(* Logix 5000 AddOnInstructionDefinition export AMCI_SV160E2_Tuning; software revision 20.03 *)

ADD_ON_INSTRUCTION AMCI_SV160E2_Tuning   (* revision 1.0, vendor AMCI, ExecuteEnableInFalse *)
// Revision note:
// 8/2019 Version 0 Initial release of SV160E2 Add On Instructions.
// 3/17/20 Version 1 replaced the generic EDS file with a more complete V1.6 EDS file.
VAR_INPUT
   Status_Word_0 : INT; {required}
        .0   // Set when the SV160E2 is moving CW
        .1   // Set when SV160E2 is moving CCW
        .7   // SV160E2 Move Complete bit
        .11   // Set when there is an input error
        .12   // set when there is a command error
        .13   // set when there is a configuration error
   Status_Word_1 : INT; {required}
        .15   // Set when SV160E2 is enabled
   Veloctiy_Loop_Proportional_Gain : INT; {required}
   Velocity_Loop_Integral_Gain : INT; {required}
   Velocity_Feedback_Low_Pass_Filter : INT; {required}
   Position_Loop_Proportional_Gain : INT; {required}
   Position_Loop_Integral_Gain : INT; {required}
   Position_Loop_Derivative_Gain : INT; {required}
   Maximim_Position_Error_Limit : INT; {required}
END_VAR
VAR_IN_OUT
   AMCI_SV160E2_output_data : _000A:SV160E2_9125ACD4:O:0; {required}
END_VAR
VAR_OUTPUT
   EN : BOOL; {access Read Only, visible}   // AOI EN bit
   DN : BOOL; {access Read Only, visible}   // AOI DN bit
   Config_ER : BOOL; {access Read Only, visible}   // AOI ER bit
   data_block_with_error : INT; {access Read Only, visible}
   data_word_with_error : INT; {access Read Only, visible}
END_VAR
VAR
   command_data_block : INT[10];
   tuning_counter : COUNTER := (PRE := 2); {access None}
END_VAR

ROUTINE EnableInFalse   (* ladder *)
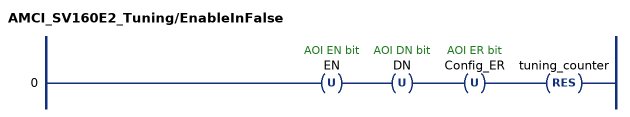
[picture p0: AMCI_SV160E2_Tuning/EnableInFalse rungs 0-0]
   0: OTU(EN)OTU(DN)OTU(Config_ER)RES(tuning_counter);
END_ROUTINE

ROUTINE Logic   (* ladder *)
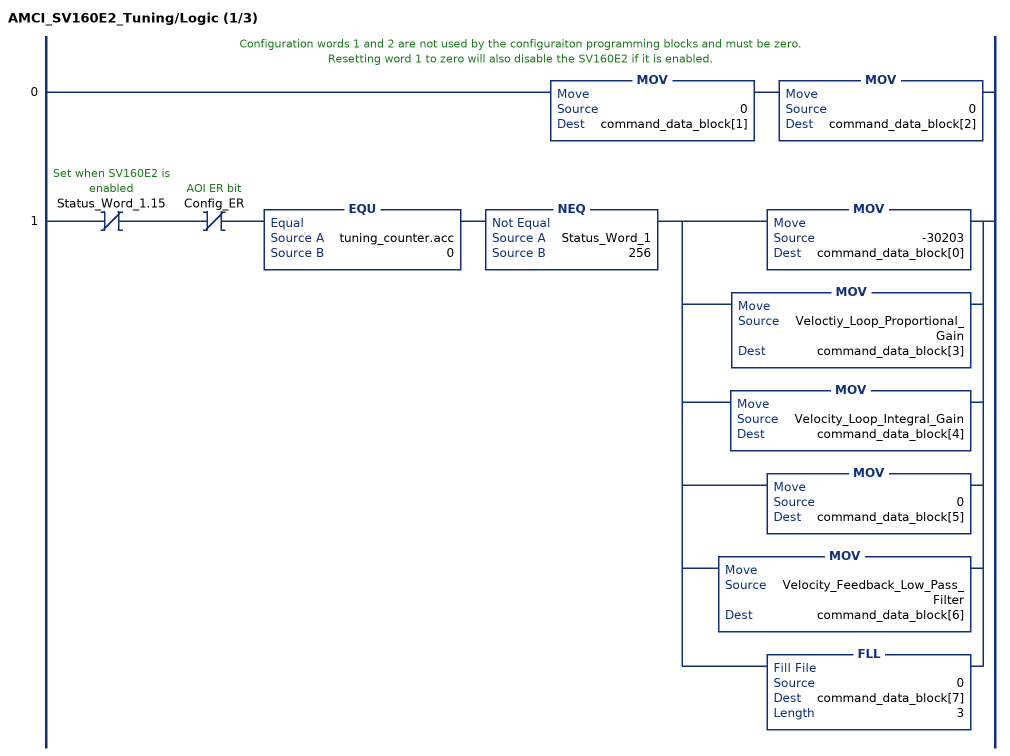
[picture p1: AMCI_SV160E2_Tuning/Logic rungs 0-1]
   // Configuration words 1 and 2 are not used by the configuraiton programming blocks and must be zero.
   // Resetting word 1 to zero will also disable the SV160E2 if it is enabled.
   0: MOV(0,command_data_block[1])MOV(0,command_data_block[2]);
   1: XIO(Status_Word_1.15)XIO(Config_ER)EQU(tuning_counter.acc,0)NEQ(Status_Word_1,256)[MOV(-30203,command_data_block[0]) ,MOV(Veloctiy_Loop_Proportional_Gain,command_data_block[3]) ,MOV(Velocity_Loop_Integral_Gain,command_data_block[4]) ,MOV(0,command_data_block[5]) ,MOV(Velocity_Feedback_Low_Pass_Filter,command_data_block[6]) ,FLL(0,command_data_block[7],3) ];
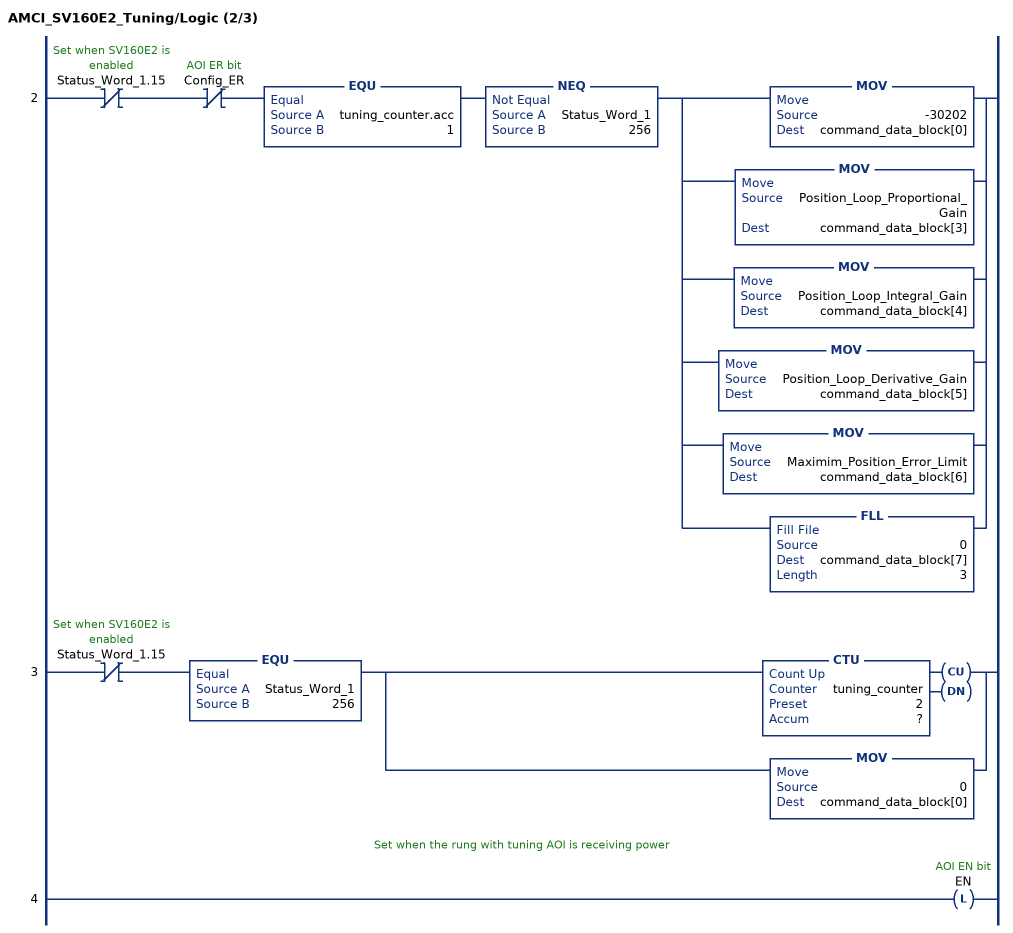
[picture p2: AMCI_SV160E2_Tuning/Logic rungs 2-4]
   2: XIO(Status_Word_1.15)XIO(Config_ER)EQU(tuning_counter.acc,1)NEQ(Status_Word_1,256)[MOV(-30202,command_data_block[0]) ,MOV(Position_Loop_Proportional_Gain,command_data_block[3]) ,MOV(Position_Loop_Integral_Gain,command_data_block[4]) ,MOV(Position_Loop_Derivative_Gain,command_data_block[5]) ,MOV(Maximim_Position_Error_Limit,command_data_block[6]) ,FLL(0,command_data_block[7],3) ];
   3: XIO(Status_Word_1.15)EQU(Status_Word_1,256)[CTU(tuning_counter,?,?) ,MOV(0,command_data_block[0]) ];
   // Set when the rung with tuning AOI is receiving power
   4: OTL(EN);
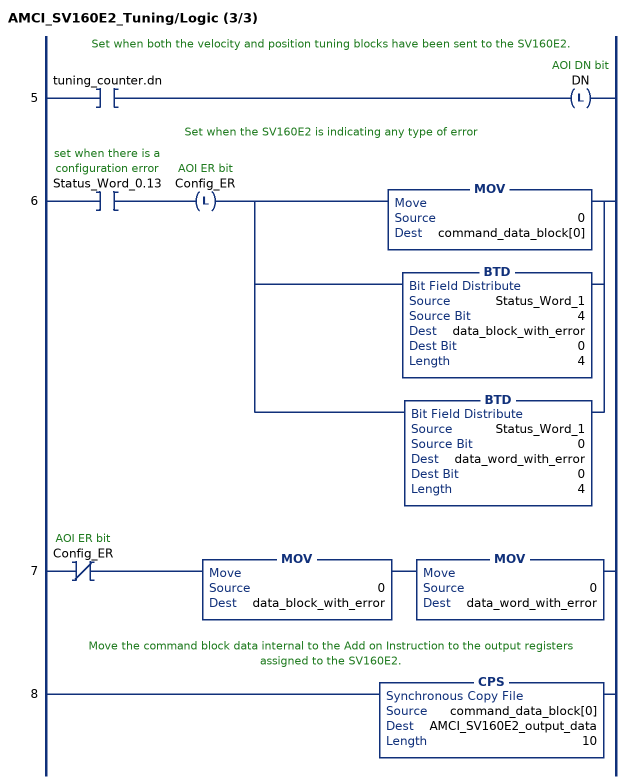
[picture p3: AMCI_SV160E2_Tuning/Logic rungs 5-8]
   // Set when both the velocity and position tuning blocks have been sent to the SV160E2.
   5: XIC(tuning_counter.dn)OTL(DN);
   // Set when the SV160E2 is indicating any type of error
   6: XIC(Status_Word_0.13)OTL(Config_ER)[MOV(0,command_data_block[0]) ,BTD(Status_Word_1,4,data_block_with_error,0,4) ,BTD(Status_Word_1,0,data_word_with_error,0,4) ];
   7: XIO(Config_ER)MOV(0,data_block_with_error)MOV(0,data_word_with_error);
   // Move the command block data internal to the Add on Instruction to the output registers assigned to the SV160E2.
   8: CPS(command_data_block[0],AMCI_SV160E2_output_data,10);
END_ROUTINE
END_ADD_ON_INSTRUCTION
